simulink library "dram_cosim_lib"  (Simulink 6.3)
undefined symbols (not defined in the file or in its folder): no_bitstream
libraries: xbsIndex_r4 x10, dram_cosim_lib x1

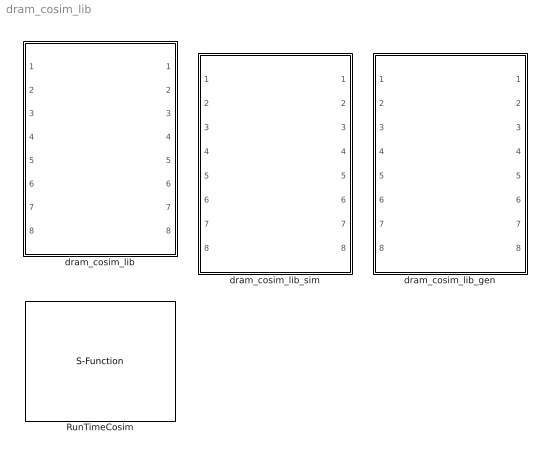
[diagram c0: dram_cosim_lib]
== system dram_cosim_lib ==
  RunTimeCosim : S-Function  FunctionName=adcosim  Parameters='d,in,unsigned,16,0;a,in,unsigned,8,0;w,in,boolean,1,0;dw,in,boolean,1,0;dr,in,boolean,1,0;q,out,unsigned,16,0;busy,out,boolean,1,0;',index,bitstream,freq,single_step,shared  mask{index=0, bitstream=no_bitstream, freq=50, single_step=off, shared=None}
      mask prompts: index "Card Index"; freq "Clock Frequency"; single_step "Single Step"; shared "Share Access"
  dram_cosim_lib : Subsystem  Tag=configX  BlockChoice=dram_cosim_lib_sim
  dram_cosim_lib_gen : Subsystem
  dram_cosim_lib_sim : Subsystem

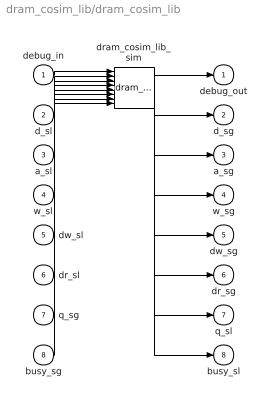
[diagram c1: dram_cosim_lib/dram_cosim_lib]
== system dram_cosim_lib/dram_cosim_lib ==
  debug_in : Inport
  d_sl : Inport  Port=2
  a_sl : Inport  Port=3
  w_sl : Inport  Port=4
  dw_sl : Inport  Port=5
  dr_sl : Inport  Port=6
  q_sg : Inport  Port=7
  busy_sg : Inport  Port=8
  dram_cosim_lib_sim : dram_cosim_lib/dram_cosim_lib_sim
  debug_out : Outport
  d_sg : Outport  Port=2
  a_sg : Outport  Port=3
  w_sg : Outport  Port=4
  dw_sg : Outport  Port=5
  dr_sg : Outport  Port=6
  q_sl : Outport  Port=7
  busy_sl : Outport  Port=8
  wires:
  debug_in/1 -> dram_cosim_lib_sim/1
  d_sl/1 -> dram_cosim_lib_sim/2
  a_sl/1 -> dram_cosim_lib_sim/3
  w_sl/1 -> dram_cosim_lib_sim/4
  dw_sl/1 -> dram_cosim_lib_sim/5
  dr_sl/1 -> dram_cosim_lib_sim/6
  q_sg/1 -> dram_cosim_lib_sim/7
  busy_sg/1 -> dram_cosim_lib_sim/8
  dram_cosim_lib_sim/1 -> debug_out/1
  dram_cosim_lib_sim/2 -> d_sg/1
  dram_cosim_lib_sim/3 -> a_sg/1
  dram_cosim_lib_sim/4 -> w_sg/1
  dram_cosim_lib_sim/5 -> dw_sg/1
  dram_cosim_lib_sim/6 -> dr_sg/1
  dram_cosim_lib_sim/7 -> q_sl/1
  dram_cosim_lib_sim/8 -> busy_sl/1

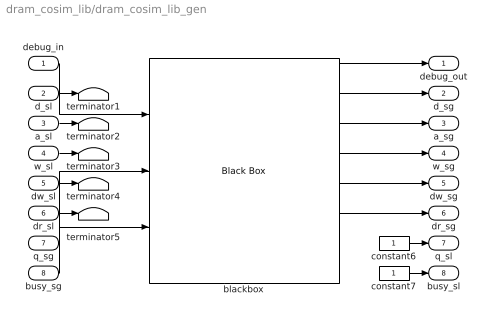
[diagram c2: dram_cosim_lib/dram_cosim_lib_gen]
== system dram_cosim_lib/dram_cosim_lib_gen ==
  debug_in : Inport
  d_sl : Inport  Port=2
  a_sl : Inport  Port=3
  w_sl : Inport  Port=4
  dw_sl : Inport  Port=5
  dr_sl : Inport  Port=6
  q_sg : Inport  Port=7
  busy_sg : Inport  Port=8
  blackbox : xbsIndex_r4/Black Box  init_code=dram_cosim_lib_config  sim_method=Inactive  block_type=blackbox2
  constant6 : Constant
  constant7 : Constant
  terminator{1..5} (5 alike) : Terminator
  debug_out : Outport
  d_sg : Outport  Port=2
  a_sg : Outport  Port=3
  w_sg : Outport  Port=4
  dw_sg : Outport  Port=5
  dr_sg : Outport  Port=6
  q_sl : Outport  Port=7
  busy_sl : Outport  Port=8
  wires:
  d_sl/1 -> terminator1/1
  a_sl/1 -> terminator2/1
  w_sl/1 -> terminator3/1
  dw_sl/1 -> terminator4/1
  dr_sl/1 -> terminator5/1
  constant6/1 -> q_sl/1
  constant7/1 -> busy_sl/1
  debug_in/1 -> blackbox/1
  blackbox/1 -> debug_out/1
  blackbox/2 -> d_sg/1
  blackbox/3 -> a_sg/1
  blackbox/4 -> w_sg/1
  blackbox/5 -> dw_sg/1
  blackbox/6 -> dr_sg/1
  q_sg/1 -> blackbox/2
  busy_sg/1 -> blackbox/3

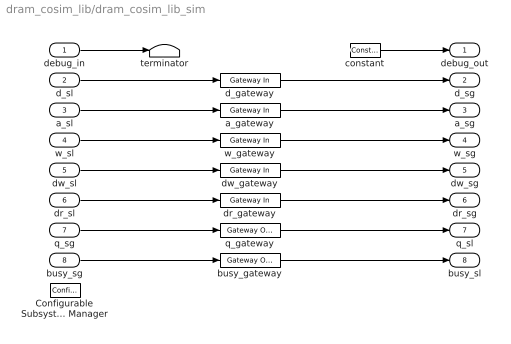
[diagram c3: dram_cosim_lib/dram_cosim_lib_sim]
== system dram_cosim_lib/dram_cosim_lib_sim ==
  debug_in : Inport
  d_sl : Inport  Port=2
  a_sl : Inport  Port=3
  w_sl : Inport  Port=4
  dw_sl : Inport  Port=5
  dr_sl : Inport  Port=6
  q_sg : Inport  Port=7
  busy_sg : Inport  Port=8
  Configurable Subsystem Manager : xbsIndex_r4/Configurable Subsystem Manager  Tag=xcfgMgr  block_type=configsubsys
  a_gateway : xbsIndex_r4/Gateway In  arith_type=Unsigned  n_bits=8  bin_pt=0  period=1  dbl_ovrd=off  timing_constraint=None  locs_specified=off  LOCs={}  block_type=gatewayin
  busy_gateway : xbsIndex_r4/Gateway Out  hdl_port=on  timing_constraint=None  locs_specified=off  LOCs={}  block_type=gatewayout
  constant : xbsIndex_r4/Constant  arith_type=Unsigned  const=1  n_bits=32  bin_pt=0  explicit_period=on  period=1  equ=P=C  opselect=C  inp2=PCIN>>17  opr=+  inp1=P  carry=CIN  dbl_ovrd=off  block_type=constant
  d_gateway : xbsIndex_r4/Gateway In  arith_type=Unsigned  n_bits=16  bin_pt=0  period=1  dbl_ovrd=off  timing_constraint=None  locs_specified=off  LOCs={}  block_type=gatewayin
  dr_gateway : xbsIndex_r4/Gateway In  arith_type=Boolean  n_bits=1  bin_pt=0  period=1  dbl_ovrd=off  timing_constraint=None  locs_specified=off  LOCs={}  block_type=gatewayin
  dw_gateway : xbsIndex_r4/Gateway In  arith_type=Boolean  n_bits=1  bin_pt=0  period=1  dbl_ovrd=off  timing_constraint=None  locs_specified=off  LOCs={}  block_type=gatewayin
  q_gateway : xbsIndex_r4/Gateway Out  hdl_port=on  timing_constraint=None  locs_specified=off  LOCs={}  block_type=gatewayout
  terminator : Terminator
  w_gateway : xbsIndex_r4/Gateway In  arith_type=Boolean  n_bits=1  bin_pt=0  period=1  dbl_ovrd=off  timing_constraint=None  locs_specified=off  LOCs={}  block_type=gatewayin
  debug_out : Outport
  d_sg : Outport  Port=2
  a_sg : Outport  Port=3
  w_sg : Outport  Port=4
  dw_sg : Outport  Port=5
  dr_sg : Outport  Port=6
  q_sl : Outport  Port=7
  busy_sl : Outport  Port=8
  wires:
  debug_in/1 -> terminator/1
  constant/1 -> debug_out/1
  d_sl/1 -> d_gateway/1
  d_gateway/1 -> d_sg/1
  a_sl/1 -> a_gateway/1
  a_gateway/1 -> a_sg/1
  w_sl/1 -> w_gateway/1
  w_gateway/1 -> w_sg/1
  dw_sl/1 -> dw_gateway/1
  dw_gateway/1 -> dw_sg/1
  dr_sl/1 -> dr_gateway/1
  dr_gateway/1 -> dr_sg/1
  q_sg/1 -> q_gateway/1
  q_gateway/1 -> q_sl/1
  busy_sg/1 -> busy_gateway/1
  busy_gateway/1 -> busy_sl/1
